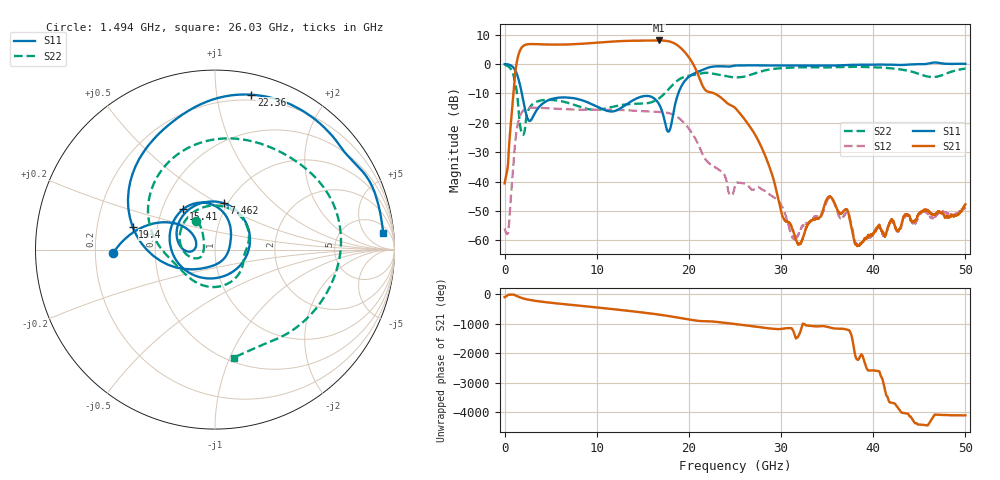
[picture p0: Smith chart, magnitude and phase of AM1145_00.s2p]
!Agilent Technologies,E8364B,MY43040894,A.07.50.67
!Agilent E8364B: A.07.50.67
!Date: Monday, November 15, 2021 11:31:16
!Correction: S11(Full 2 Port(1,2))
!S21(Full 2 Port(1,2))
!S12(Full 2 Port(1,2))
!S22(Full 2 Port(1,2))
!S2P File: Measurements: S11, S21, S12, S22:
# Hz S  dB  R 50
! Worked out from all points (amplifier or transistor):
!   6401 points, 10 MHz to 50 GHz, reference 50 ohm
!   highest |S21| = 8.0 dB at 16.71 GHz (marker M1)
!   |S21| within 3 dB of that: 1.745 GHz to 19.27 GHz (17.52 GHz wide, 167 % of centre)
!   unconditionally stable (mu >= 1): start of sweep to 45.76 GHz
!   at 8.336 GHz: K = 1.42, MAG = 7.4 dB, |S12| = -15.5 dB
!   at 25 GHz: K = 25.21, MAG = -3.9 dB, |S12| = -41.2 dB
!   at 50 GHz: K = -111.91, MSG = 0.8 dB, |S12| = -49.3 dB
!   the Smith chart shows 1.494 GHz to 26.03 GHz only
!   S11 on the Smith chart (normalised r, x): 1.494 GHz: 0.27, -0.02; 7.462 GHz: 0.96, +0.53; 15.41 GHz: 0.64, +0.31; 19.4 GHz: 0.36, +0.12; 22.36 GHz: 0.15, +1.25; 26.03 GHz: 9, +15
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1e7  -0.05 -12.6  -40.61 -94.3  -55.92 -114.0  -0.26 -16.8
8.84825e8  -0.96 -106.7  -12.88 -5.6  -36.89 -145.3  -3.00 -143.4
1.494078e9  -4.90 -177.8  2.90 -77.2  -19.67 134.9  -14.44 123.5
2.587609e9  -19.09 160.6  6.72 -178.8  -14.98 25.3  -15.72 -171.5
4.368503e9  -12.97 161.3  6.64 99.0  -14.99 -59.4  -12.23 105.0
7.461634e9  -11.61 78.8  6.70 -3.2  -15.49 -156.8  -13.79 22.2
8.34427e9  -12.28 55.1  6.86 -30.7  -15.54 178.0  -14.70 7.3
1.053914e10  -15.21 -18.3  7.36 -100.4  -15.57 115.2  -15.40 -20.3
1.265591e10  -14.93 -123.3  7.78 -171.6  -15.65 52.1  -13.98 -63.3
1.540536e10  -10.85 128.1  7.94 88.4  -16.12 -35.2  -13.38 -139.8
1.667854e10  -13.24 79.3  8.00 36.8  -16.28 -80.4  -11.88 -168.1
1.670978e10  -13.40 77.9  8.00 35.5  -16.29 -81.6  -11.82 -168.8
1.785018e10  -22.88 -52.8  7.68 -18.4  -16.73 -129.5  -8.41 161.2
1.939675e10  -6.45 164.5  4.58 -101.1  -19.75 154.7  -4.52 101.0
2.235709e10  -1.04 76.8  -9.62 164.2  -34.13 54.9  -3.14 -2.4
2.5005e10  -0.55 25.3  -14.91 74.9  -41.21 10.9  -4.55 -64.5
2.602823e10  -0.52 5.6  -18.72 32.0  -40.70 -42.9  -4.27 -80.1
3.176146e10  -0.51 -87.5  -60.71 -23.8  -58.65 -104.6  -1.17 -178.4
3.333927e10  -0.56 -110.9  -53.17 3.7  -52.73 41.0  -1.09 160.5
4.167354e10  -0.23 157.3  -54.96 -4.9  -54.92 -114.0  -1.37 65.9
4.659443e10  0.50 125.8  -51.18 -161.8  -52.06 -133.5  -4.44 -86.3
5e10  0.04 103.5  -47.74 -152.5  -49.30 162.2  -1.60 151.2
